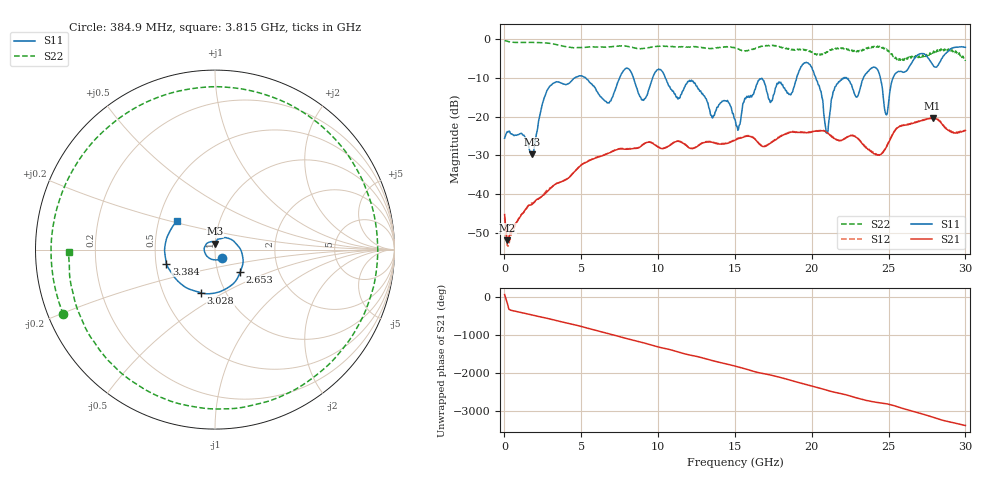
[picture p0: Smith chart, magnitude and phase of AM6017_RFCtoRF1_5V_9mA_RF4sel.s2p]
!Agilent Technologies,E8364B,MY43040894,A.07.50.67
!Agilent E8364B: A.07.50.67
!Date: Tuesday, August 21, 2018 13:36:06
!Correction: S11(Full 2 Port(1,2))
!S21(Full 2 Port(1,2))
!S12(Full 2 Port(1,2))
!S22(Full 2 Port(1,2))
!S2P File: Measurements: S11, S21, S12, S22:
# Hz S  dB  R 50
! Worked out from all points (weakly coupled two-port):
!   1601 points, 10 MHz to 30 GHz, reference 50 ohm
!   highest |S21| = -20.48 dB at 27.86 GHz (marker M1); lowest = -52.0 dB at 178.7 MHz (marker M2)
!   lowest |S11| = -29.8 dB at 1.772 GHz (marker M3), VSWR 1.07, Z = 49.9 + j3.24 ohm
!   |S11| at or under -10 dB: start of sweep to 4.587 GHz; 5.276 GHz to 7.493 GHz (2.217 GHz wide, 34.7 % of centre); 10.46 GHz to 19.02 GHz (8.554 GHz wide, 58 % of centre)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
!   |S22| runs from -5.6 to -0.3 dB; largest |S21 - S12| = 0.0086
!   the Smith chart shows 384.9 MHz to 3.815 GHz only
!   S11 on the Smith chart (normalised r, x): 384.9 MHz: 1.08, -0.10; 2.653 GHz: 1.28, -0.33; 3.028 GHz: 0.76, -0.39; 3.384 GHz: 0.57, -0.10; 3.815 GHz: 0.63, +0.21
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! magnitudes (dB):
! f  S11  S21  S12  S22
! 10 MHz  -25.6  -45.3  -46.1  -0.3
! 178.7 MHz  -23.9  -52.0  -53.3  -0.5
! 384.9 MHz  -24.3  -49.8  -51.3  -0.7
! 1.772 GHz  -29.8  -42.8  -42.3  -0.8
! 2.653 GHz  -14.5  -39.9  -39.6  -1.0
! 3.028 GHz  -11.9  -38.5  -38.4  -1.1
! 3.384 GHz  -11.0  -37.3  -37.3  -1.4
! 3.815 GHz  -11.6  -36.7  -36.6  -1.8
! 5.015 GHz  -9.4  -32.5  -32.4  -2.2
! 6.758 GHz  -16.4  -29.5  -29.5  -2.0
! 7.864 GHz  -7.7  -28.4  -28.3  -1.8
! 10.02 GHz  -7.8  -27.9  -27.8  -1.9
! 15.01 GHz  -20.8  -26.1  -25.9  -2.3
! 16.64 GHz  -10.2  -27.3  -27.2  -2.0
! 17.33 GHz  -16.3  -26.8  -26.7  -1.7
! 20.01 GHz  -7.4  -24.0  -23.9  -3.3
! 20.97 GHz  -24.3  -24.1  -23.9  -3.2
! 22.09 GHz  -10.0  -25.8  -25.8  -2.5
! 24.13 GHz  -7.3  -29.8  -29.6  -2.0
! 25.01 GHz  -15.9  -26.7  -26.5  -3.1
! 27.86 GHz  -6.5  -20.5  -20.3  -3.6
! 30 GHz  -2.1  -23.6  -23.6  -5.6
